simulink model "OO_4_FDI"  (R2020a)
settings: Solver=VariableStepAuto  StartTime=0.0  StopTime=30  RelTol=1e-3
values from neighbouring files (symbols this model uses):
  Ao1 = Am - H1*Cm(1,:)    [design_OO.m]
  Ao2 = Am - H2*Cm(2,:)    [design_OO.m]
  Bo1 = [Bm H1]    [design_OO.m]
  Bo2 = [Bm H2]    [design_OO.m]
  C = 6.3000e-04    (= 0.00063)    [maglev_init.m]
  Co1 = Cm(1,:)    [design_OO.m]
  Co2 = Cm(2,:)    [design_OO.m]
  Do1 = zeros(1,2)    [design_OO.m]
  Do2 = zeros(1,2)    [design_OO.m]
  g = 9.80    (= 9.8)    [maglev_init.m]
  K = 1.0e+03 * [-2.4567   -0.1235    0.0237]    [maglev_init.m]
  L1 = 0.6000    (= 0.6)    [maglev_init.m]
  m = 0.0300    (= 0.03)    [maglev_init.m]
  mpert = 0    [maglev_init.m]
  R = 45    [maglev_init.m]
  Ts = 0.005    [maglev_init.m]    (also in train_net.m)
  x1_0 = 0.1    [maglev_init.m]
  x1_d = 0.05    [maglev_init.m]
  x2_0 = 0    [maglev_init.m]
  x2_d = 0    [maglev_init.m]
  x3_0 = 0.2    [maglev_init.m]

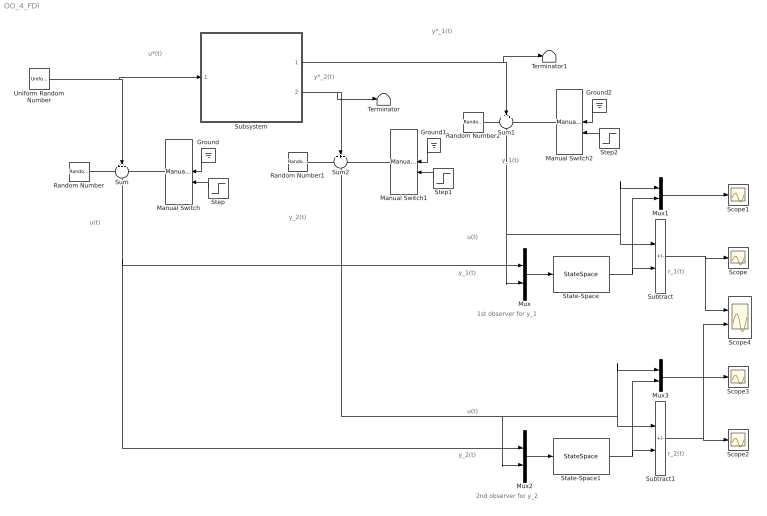
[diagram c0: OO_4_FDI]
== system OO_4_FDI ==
  note: r_1(t)
  note: u(t)
  note: 1st observer for y_1
  note: y_2(t)
  note: y*_1(t)
  note: u(t)
  note: u*(t)
  note: y*_2(t)
  note: y_1(t)
  note: y_1(t)
  note: u(t)
  note: r_2(t)
  note: y_2(t)
  note: 2nd observer for y_2
  Ground : Ground
  Ground1 : Ground
  Ground2 : Ground
  Manual Switch : ManualSwitch  CurrentSetting=0
  Manual Switch1 : ManualSwitch
  Manual Switch2 : ManualSwitch
  Mux{,1..3} (4 alike) : Mux  Inputs=2
  Random Number : RandomNumber  Variance=1e-9  Seed=1  SampleTime=Ts
  Random Number1 : RandomNumber  Variance=1e-6  Seed=3  SampleTime=Ts
  Random Number2 : RandomNumber  Variance=1e-9  Seed=2  SampleTime=Ts
  Scope{,1..3} (4 alike) : Scope
  Scope4 : Scope  NumInputPorts=2
  State-Space : StateSpace  A=Ao1  B=Bo1  C=Co1  D=Do1  InitialCondition=0
  State-Space1 : StateSpace  A=Ao2  B=Bo2  C=Co2  D=Do2  InitialCondition=0
  Step : Step  Time=15  SampleTime=0
  Step1 : Step  Time=15  SampleTime=0
  Step2 : Step  Time=15  SampleTime=0
  Subsystem : Subsystem
  Subtract : Sum  Inputs=+-
  Subtract1 : Sum  Inputs=+-
  Sum : Sum  Inputs=+++
  Sum1 : Sum  Inputs=+++
  Sum2 : Sum  Inputs=+++
  Terminator : Terminator
  Terminator1 : Terminator
  Uniform Random Number : UniformRandomNumber  Minimum=x1_d*0.9  Maximum=x1_d*1.1  Seed=1  SampleTime=0.5
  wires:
  Uniform Random Number/1 -> Subsystem/1(In1), Sum/2
  Subsystem/1(Out1) -> Terminator1/1, Sum1/2
  Subsystem/2(Out2) -> Terminator/1, Sum2/2
  Random Number/1 -> Sum/1
  Manual Switch/1 -> Sum/3
  Manual Switch2/1 -> Sum1/3
  Manual Switch1/1 -> Sum2/3
  Random Number1/1 -> Sum2/1
  Ground/1 -> Manual Switch/1
  Step/1 -> Manual Switch/2
  Ground1/1 -> Manual Switch1/1
  Step1/1 -> Manual Switch1/2
  Random Number2/1 -> Sum1/1
  Ground2/1 -> Manual Switch2/1
  Step2/1 -> Manual Switch2/2
  Sum1/1 -> Mux1/1, Subtract/1, Mux/2
  Mux/1 -> State-Space/1
  State-Space/1 -> Mux1/2, Subtract/2
  Subtract/1 -> Scope4/1, Scope/1
  Mux1/1 -> Scope1/1
  Mux3/1 -> Scope3/1
  Mux2/1 -> State-Space1/1
  Sum2/1 -> Mux2/2, Mux3/1, Subtract1/1
  Subtract1/1 -> Scope4/2, Scope2/1
  Sum/1 -> Mux2/1, Mux/1
  State-Space1/1 -> Mux3/2, Subtract1/2

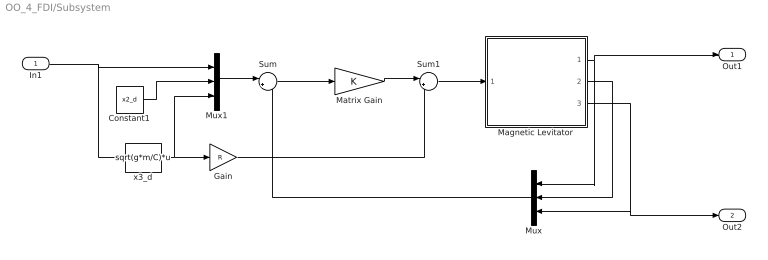
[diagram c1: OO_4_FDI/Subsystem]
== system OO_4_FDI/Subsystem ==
  In1 : Inport
  Constant1 : Constant  Value=x2_d
  Gain : Gain  Gain=R
  Magnetic Levitator : Subsystem  mask{m=m+mpert, R=R, L1=L1, C=C, g=g}
      mask prompts: m "ball's mass (m)"; R "Electromagnet's resistance (R)"; L1 "Electromagnet's inductance (L1)"; C "Magnetic force constant (C)"; g "Gravitational acceleration (g)"
  Matrix Gain : Gain  Gain=K  Multiplication=Matrix(K*u)  SaturateOnIntegerOverflow=on
  Mux : Mux  Inputs=3
  Mux1 : Mux  Inputs=3
  Sum : Sum  Inputs=|+-  InputSameDT=on  SaturateOnIntegerOverflow=on
  Sum1 : Sum  Inputs=|++  InputSameDT=on  SaturateOnIntegerOverflow=on
  x3_d : Fcn  Expr=sqrt(g*m/C)*u
  Out1 : Outport
  Out2 : Outport  Port=2
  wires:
  In1/1 -> x3_d/1, Mux1/1
  Magnetic Levitator/2(x2) -> Mux/2
  x3_d/1 -> Mux1/3, Gain/1
  Mux1/1 -> Sum/1
  Gain/1 -> Sum1/2
  Mux/1 -> Sum/2
  Constant1/1 -> Mux1/2
  Sum/1 -> Matrix Gain/1
  Sum1/1 -> Magnetic Levitator/1(u)
  Magnetic Levitator/1(x1) -> Out1/1, Mux/1
  Magnetic Levitator/3(x3) -> Out2/1, Mux/3
  Matrix Gain/1 -> Sum1/1

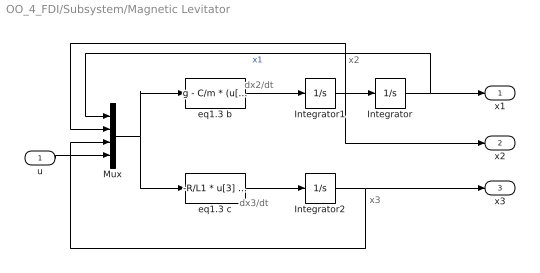
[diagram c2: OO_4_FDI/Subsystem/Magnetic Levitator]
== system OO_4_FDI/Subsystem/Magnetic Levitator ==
  note: x2
  note: x3
  note: dx2/dt
  note: dx3/dt
  u : Inport
  Integrator : Integrator  InitialCondition=x1_0
  Integrator1 : Integrator  InitialCondition=x2_0
  Integrator2 : Integrator  InitialCondition=x3_0
  Mux : Mux
  eq1.3 b : Fcn  Expr=g - C/m * (u[3] / u[1])^2
  eq1.3 c : Fcn  Expr=-R/L1 * u[3] + (2*C)/L1 * ( u[2] * u[3] / u[1]^2 ) + 1/L1 * u[4]
  x1 : Outport
  x2 : Outport  Port=2
  x3 : Outport  Port=3
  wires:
  eq1.3 b/1 -> Integrator1/1
  Integrator1/1 -> Integrator/1, Mux/2, x2/1
  eq1.3 c/1 -> Integrator2/1
  Mux/1 -> eq1.3 b/1, eq1.3 c/1
  Integrator/1 -> Mux/1, x1/1  "x1"
  Integrator2/1 -> Mux/3, x3/1
  u/1 -> Mux/4
